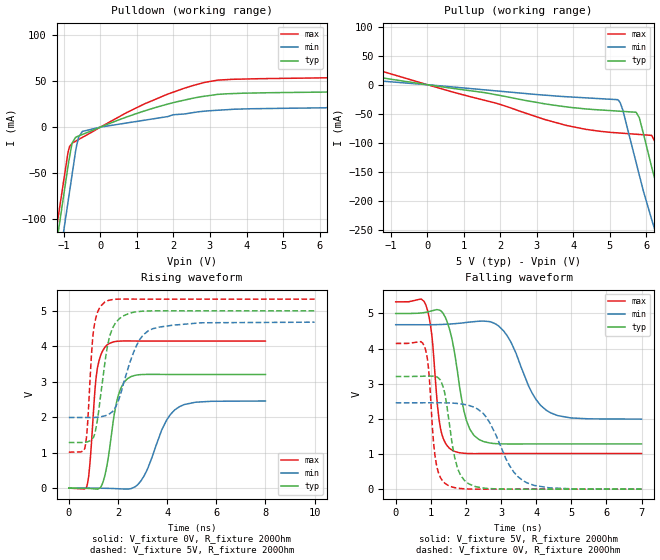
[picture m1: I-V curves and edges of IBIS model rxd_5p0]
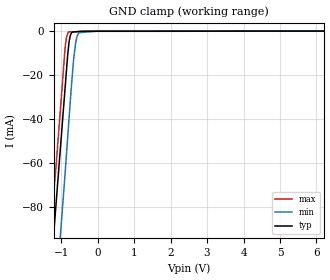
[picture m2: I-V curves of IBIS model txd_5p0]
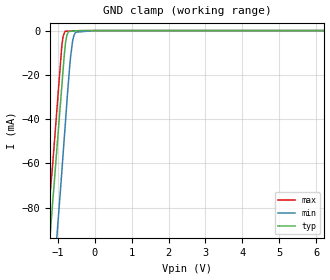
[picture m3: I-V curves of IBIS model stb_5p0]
| Texas Instruments Incorporated
| 5-V CAN TRANSCEIVER WITH I/O LEVEL ADAPTING AND LOW-POWER MODE SUPPLY
| OPTIMIZATION
| Marketing part#   Digital Voltage Range   Package-type   #pins
| HVDA553QDRQ1   3V-5.33V   SOIC-D   8
[IBIS Ver]   4.1
[File name]   hvda553.ibs
[File Rev]   1.0
[Date]   5/30/2013
[Source]
| Texas Instruments Incorporated.
| Analog-eLab Design Center, HPA
| 12500 TI Blvd
| Dallas, TX -75243
[Notes]   Revision History:
| Rev 1.0: 5/30/2013
| - Initial version of the model
| - Model generated from simulations in TISPICE
| - Model matched to SPICE simulation
| - C_comp although listed in numerical order of value are
|   obtained from varying PVT conditions. For PVT conditions for
|   each specific value refer the buffer description under
|   respective [Model]. IBIS model user is responsible for using
|   appropriate C_comp to simulate for Signal Integrity.
| - Relative part of HVDA551 .
| - SPLIT buffer is modelled for HVDA553.
[Disclaimer]
| This model is designed as an aid for customers of Texas Instruments.
| TI and its licensors and suppliers make no warranties, either expressed
| or implied, with respect to this  model, including the warranties of
| merchantability or fitness for a particular purpose. The model is
| provided solely on an "as is" basis. The entire risk as to its quality
| and performance is with the customer.
[Copyright]
(C) Copyright 2013 Texas Instruments Incorporated.All rights reserved.
|   HVDA553
[Component]   HVDA553
[Manufacturer]   TI
[Package]   |8-SOIC   -  D package
|   typ   min   max
R_pkg   0.127685   0.11951   0.13703
L_pkg   2.762815nH   2.62615nH   2.93615nH
C_pkg   0.3886967pF  0.37236pF   0.40249pF
[Pin]  signal_name   model_name   R_pin   L_pin   C_pin
1   TXD   txd_5p0   0.11951   2.62615nH  0.38237pF
2   GND   gnd   0.05984   2.09355nH  0.43647pF
3   VCC   power   0.05549   1.98027nH  0.42953pF
4   RXD   rxd_5p0   0.11969   2.67863nH  0.37236pF
5   SPLIT   split   0.13694   2.93615nH  0.38275pF
6   CANL   can_l   0.13062   2.78789nH  0.40249pF
7   CANH   can_h   0.12232   2.66240nH  0.39769pF
8   STB   stb_5p0   0.13703   2.88567nH  0.39452pF
[Diff_pin]   inv_pin   vdiff   tdelay_typ   tdelay_min   tdelay_max
7   6   500mV   NA   NA   NA
|   Model Selectors
[Model Selector] can_h
can_input_p 5.0V differential input  [Standby_mode]
canh_os   5.0V I/O_open_source   [Normal_mode]
[Model Selector] can_l
can_input_n 5.0V differential input  [Standby_mode]
canl_od   5.0V I/O_open_drain   [Normal_mode]
| Models and submodels in the file (8): rxd_5p0 (Output), txd_5p0 (Input), stb_5p0 (Input), canh_os (I/O_open_source), canl_od (I/O_open_drain), can_input_p (Input), can_input_n (Input), split (3-state)
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|   rxd_5p0 Model
[Model]   rxd_5p0
Model_type   Output
Polarity   Non-Inverting
Vmeas = 2.5
Vref = 0
Cref = 15pF
Rref = 400
|   typ   min   max
|   (nom PVT)   (fast PVT)   (slow PVT)
C_comp   1.031e-12   7.804e-13   1.060e-12
| Where nom  PVT is Nominal Process, 5V, 27C
|   Fast PVT is Strong Process,  5.33V, -40C
|   Slow PVT is Weak Process,   4.68V, 150C
[Voltage Range]   5   4.68   5.33
|Junction Temperature
[Temperature Range]   27   150   -40
[Pullup Reference]   5   4.68   5.33
[Pulldown Reference]   0   0   0
[Power Clamp Reference]   5   4.68   5.33
[GND Clamp Reference]   0   0   0
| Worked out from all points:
|   slope of the pulldown table from 0 to 0.75 V, typ, clamps not added: 65.7 ohm
|   slope of the pullup table from 0 to 0.75 V, typ, clamps not added: 111 ohm
|   falling waveform, V_fixture 5V, R_fixture 200Ohm: 20-80 % time 388ps typ, 711ps min, 234ps max; typ from 5 V to 1.29 V
|   rising waveform, V_fixture 0V, R_fixture 200Ohm: 20-80 % time 440ps typ, 855ps min, 274ps max; typ from 0 V to 3.21 V
|   rising waveform, V_fixture 5V, R_fixture 200Ohm: 20-80 % time 468ps typ, 802ps min, 241ps max; typ from 1.29 V to 5 V
|   falling waveform, V_fixture 0V, R_fixture 200Ohm: 20-80 % time 322ps typ, 729ps min, 193ps max; typ from 3.21 V to 0 V
[Pulldown]
|   Voltage   I(typ)   I(min)   I(max)
-5V       -897.3mA   -876.2mA   -949.2mA
-1.327V   -160mA     -193.3mA   -142.6mA
-1.104V   -100.7mA   -139mA     -84.37mA
-1.067V   -90.73mA   -129.4mA   -74.57mA
-879.4mV  -40.8mA    -79.54mA   -26.35mA
-775mV    -17.44mA   -51.74mA   -17.75mA
-650.5mV  -10.45mA   -20.08mA   -14.65mA
-491.4mV  -7.891mA   -4.616mA   -11.11mA
2.526V    31.27mA    15.67mA    44.96mA
6.668V    38.91mA    23.78mA    53.72mA
9.36V     76.66mA    43.65mA    116mA
10V       86.67mA    48.38mA    132.6mA
[Pullup]
|   Voltage   I(typ)   I(min)   I(max)
-5V       56.18mA    31.7mA     97.1mA
3.209V    -32.8mA    -17.94mA   -59.75mA
5.214V    -45.37mA   -25.77mA   -82.88mA
5.359V    -45.95mA   -44.77mA   -83.55mA
5.71V     -47.37mA   -132mA     -85.16mA
5.805V    -56.73mA   -155.5mA   -85.61mA
6.14V     -140.9mA   -231.2mA   -87.2mA
6.231V    -162.1mA   -249.7mA   -97.78mA
6.618V    -244.8mA   -328.5mA   -189.8mA
6.675V    -256.1mA   -340.2mA   -202.9mA
6.972V    -316.8mA   -398.7mA   -261.7mA
10V       -897.6mA   -929.7mA   -883.7mA
[Ramp]
R_load = 200
|   typ   min   max
dV/dt_r   1.92355/4.39108e-10   1.47461/8.50569e-10   2.48848/2.73295e-10
dV/dt_f   2.2278/3.85654e-10   1.61217/7.06838e-10   2.58905/2.32122e-10
[Falling Waveform]
V_fixture = 5V
V_fixture_min = 4.68V
V_fixture_max = 5.33V
R_fixture = 200Ohm
|   Time   V(typ)   V(min)   V(max)
0s        5V         4.68V      5.33V
860ps     5.034V     4.679V     5.239V
1.028ns   5.075V     4.68V      4.39V
1.274ns   5.083V     4.686V     1.741V
1.604ns   4.269V     4.704V     1.111V
2.012ns   1.963V     4.744V     1.016V
2.362ns   1.419V     4.778V     1.012V
3.068ns   1.287V     4.509V     1.015V
4.408ns   1.287V     2.174V     1.015V
6.998ns   1.287V     1.993V     1.015V
[Rising Waveform]
V_fixture = 0V
V_fixture_min = 0V
V_fixture_max = 0V
R_fixture = 200Ohm
|   Time   V(typ)   V(min)   V(max)
0s        442pV      23.7nV     378.5pV
734ps     -6.129mV   327.4uV    49.78mV
858ps     -10.35mV   94.12uV    690.2mV
1.15ns    -28.2mV    -1.545mV   3.327V
1.384ns   156.1mV    -3.822mV   3.882V
1.598ns   829.7mV    -6.605mV   4.059V
1.998ns   2.582V     -16.57mV   4.143V
2.536ns   3.147V     -11.83mV   4.15V
4.508ns   3.206V     2.3V       4.147V
7.998ns   3.206V     2.458V     4.147V
[Rising Waveform]
V_fixture = 5V
V_fixture_min = 4.68V
V_fixture_max = 5.33V
R_fixture = 200Ohm
|   Time   V(typ)   V(min)   V(max)
0s        1.287V     1.993V     1.015V
646ps     1.292V     1.991V     1.11V
756ps     1.306V     1.991V     1.739V
1.006ns   1.437V     1.992V     4.448V
1.46ns    3.496V     2.037V     5.245V
1.682ns   4.327V     2.108V     5.306V
2.02ns    4.754V     2.476V     5.33V
2.752ns   4.974V     4.017V     5.331V
3.404ns   4.999V     4.492V     5.33V
9.998ns   5V         4.68V      5.33V
[Falling Waveform]
V_fixture = 0V
V_fixture_min = 0V
V_fixture_max = 0V
R_fixture = 200Ohm
|   Time   V(typ)   V(min)   V(max)
0s        3.206V     2.458V     4.147V
822ps     3.215V     2.458V     4.059V
934ps     3.217V     2.459V     3.438V
1.068ns   3.214V     2.459V     1.45V
1.156ns   3.201V     2.459V     718.5mV
1.462ns   2.34V      2.455V     124.5mV
1.758ns   609.3mV    2.438V     28.51mV
2.236ns   83.11mV    2.332V     552.5uV
3.742ns   213.1uV    177.7mV    -15.95uV
6.998ns   -18.92nV   316.2nV    -66.52nV
|   txd_5p0 Model
[Model]   txd_5p0
Model_type   Input
Vinl = 1.5
Vinh = 3.5
|   typ   min   max
|   (nom PVT)   (fast PVT)   (slow PVT)
C_comp   3.681e-13   3.534e-13   3.972e-13
[Model spec]
|subparameter
Vinl   1.5   1.404   1.533
Vinh   3.5   3.276   3.731
| Where nom  PVT is Nominal Process, 5V, 27C
|   Fast PVT is Strong Process,  5.33V, -40C
|   Slow PVT is Weak Process,   4.68V, 150C
[Voltage Range]   5   4.68   5.33
|Junction Temperature
[Temperature Range]   27   150   -40
[Power Clamp Reference]   5   4.68   5.33
[GND Clamp Reference]   0   0   0
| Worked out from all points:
|   GND clamp passes 1 mA (typ) near -0.72 V on its own axis
[GND Clamp]
|   Voltage   I(typ)   I(min)   I(max)
-5V       -570.8mA   -621mA     -524.6mA
-1.327V   -118.4mA   -152.3mA   -97.06mA
-1.179V   -87.06mA   -125mA     -68.94mA
-1.03V    -55.26mA   -94.85mA   -37.66mA
-879.4mV  -23.38mA   -61.88mA   -5.934mA
-852.8mV  -17.65mA   -55.78mA   -2.672mA
-799.5mV  -7.615mA   -43.59mA   -361.9uA
-750mV    -2.038mA   -32.27mA   -340.1uA
-650.5mV  -391.2uA   -11.93mA   -296.4uA
-594.4mV  -306.8uA   -4.637mA   -271.7uA
-514.8mV  -187.3uA   -745.1uA   -236.7uA
10V       0A         0A         0A
[POWER Clamp]
|   Voltage   I(typ)   I(min)   I(max)
-5V       0A         0A         0A
0V        0A         0A         0A
10V       0A         0A         0A
|   stb_5p0 Model
[Model]   stb_5p0
Model_type   Input
Vinl = 1.5
Vinh = 3.5
|   typ   min   max
|   (nom PVT)   (fast PVT)   (slow PVT)
C_comp   3.681e-13   3.534e-13   3.972e-13
[Model spec]
|subparameter
Vinl   1.5   1.404   1.533
Vinh   3.5   3.276   3.731
| Where nom  PVT is Nominal Process, 5V, 27C
|   Fast PVT is Strong Process,  5.33V, -40C
|   Slow PVT is Weak Process,   4.68V, 150C
[Voltage Range]   5   4.68   5.33
|Junction Temperature
[Temperature Range]   27   150   -40
[Power Clamp Reference]   5   4.68   5.33
[GND Clamp Reference]   0   0   0
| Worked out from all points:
|   GND clamp passes 1 mA (typ) near -0.72 V on its own axis
[GND Clamp]
|   Voltage   I(typ)   I(min)   I(max)
-5V       -570.8mA   -621mA     -524.6mA
-1.327V   -118.4mA   -152.3mA   -97.03mA
-1.179V   -87.05mA   -125mA     -68.91mA
-1.03V    -55.25mA   -94.85mA   -37.62mA
-879.4mV  -23.36mA   -61.87mA   -5.88mA
-852.8mV  -17.63mA   -55.78mA   -2.614mA
-799.5mV  -7.587mA   -43.59mA   -296.2uA
-750mV    -2.004mA   -32.27mA   -271.8uA
-650.5mV  -348.6uA   -11.92mA   -222.9uA
-594.4mV  -261.8uA   -4.628mA   -195.3uA
-514.8mV  -138.9uA   -731.7uA   -156.2uA
10V       0A         0A         0A
[POWER Clamp]
|   Voltage   I(typ)   I(min)   I(max)
-5V       0A         0A         0A
0V        0A         0A         0A
10V       0A         0A         0A
